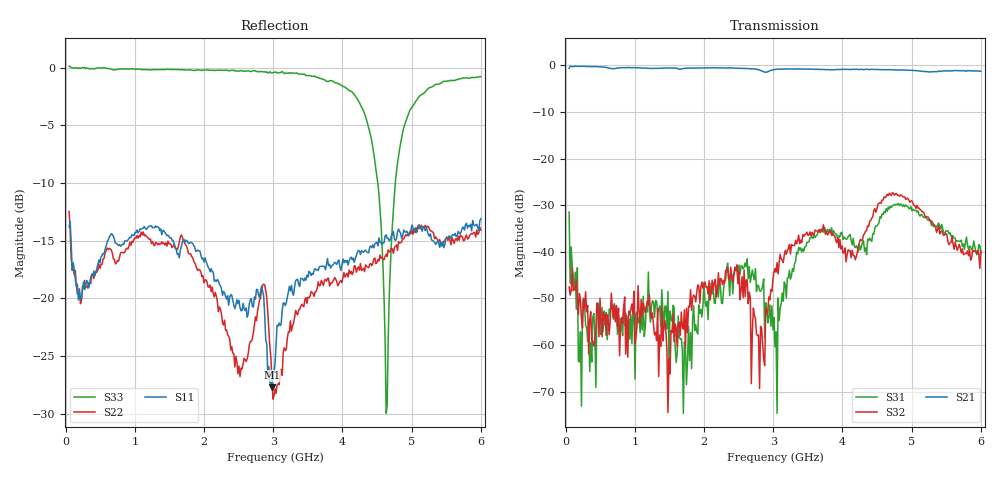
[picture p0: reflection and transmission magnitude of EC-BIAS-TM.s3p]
! MDIF file - written using SXPWrite.m
# GHz S RI R 50
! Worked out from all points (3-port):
!   401 points, 50 MHz to 6 GHz, reference 50 ohm
!   strongest paths, dB at 50 MHz, 1.538 GHz, 3.025 GHz, 4.513 GHz, 6 GHz:
!     S21: -0.6, -0.6, -0.9, -0.9, -1.3
!     S32: -47.5, -57.3, -43.6, -29.8, -39.8
!     S31: -31.5, -54.9, -60.4, -34.1, -40.3
!   lowest |S11| = -27.7 dB at 2.98 GHz (marker M1), VSWR 1.09, Z = 49.4 - j4.06 ohm
!   |S11| at or under -10 dB: start of sweep to end of sweep
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0.05  0.0696 -0.1917  0.9158 0.2787  0.0137 -0.0111
      0.8873 0.2859  0.121 -0.2051  -0.0159 0.0172
      0.0219 -0.0152  0.00404 -0.00113  -1.016 -0.0236
0.213625  -0.0258 -0.0952  0.95 -0.2508  -0.000804 -0.000298
          0.9436 -0.2462  -0.0295 -0.0901  0.000941 -0.0003
          0.00136 0.00027  0.00174 0.00251  -0.9655 0.2378
1.076375  -0.1961 0.0412  -0.0956 -0.9409  -0.000616 0.00176
          -0.093 -0.9383  -0.182 0.033  0.00152 0.00354
          0.000262 0.00134  0.00119 0.00123  -0.3323 0.9303
2.028375  0.0571 0.1331  -0.9468 -0.00354  0.000241 0.00182
          -0.9387 -0.00305  -0.0205 0.1185  0.005 0.00156
          0.00223 0.00135  0.0039 0.00144  0.7425 0.6382
2.980375  -0.00389 -0.0409  -0.1141 0.8898  2.38e-05 0.000641
          -0.1111 0.8842  0.0176 0.0409  0.0051 -9.15e-05
          -0.00222 -0.00143  0.00257 -0.00274  0.744 -0.5911
3.025  -0.00905 -0.0507  -0.0471 0.9083  -0.000122 -0.00125
       -0.0487 0.9013  0.0046 0.0403  0.00559 -0.00263
       -0.000358 0.000885  0.00597 -0.0029  0.7098 -0.6403
4.170375  -0.1211 0.077  0.8934 -0.1773  -0.0024 0.0106
          0.8893 -0.1789  0.1385 0.00733  -0.00679 0.00281
          0.000113 0.0114  -0.00773 0.00473  -0.6939 -0.3251
4.6315  -0.0986 0.1606  0.5406 -0.7259  0.0173 0.0224
        0.5366 -0.7188  0.0857 -0.1298  0.00346 0.0391
        0.0171 0.0234  0.00203 0.0393  -0.0317 0.00259
4.914125  -0.0338 0.1906  0.1712 -0.8761  0.0279 -0.0167
          0.1647 -0.875  -0.00555 -0.1889  0.0361 0.00219
          0.0287 -0.014  0.0363 0.00348  -0.2876 -0.5089
6  0.2213 -0.013  -0.8685 -0.048  -0.0129 -0.000615
   -0.8642 -0.0462  -0.1973 0.0142  -0.00548 -0.00898
   -0.00965 -9.92e-05  -0.00757 -0.00683  -0.5386 0.7386
